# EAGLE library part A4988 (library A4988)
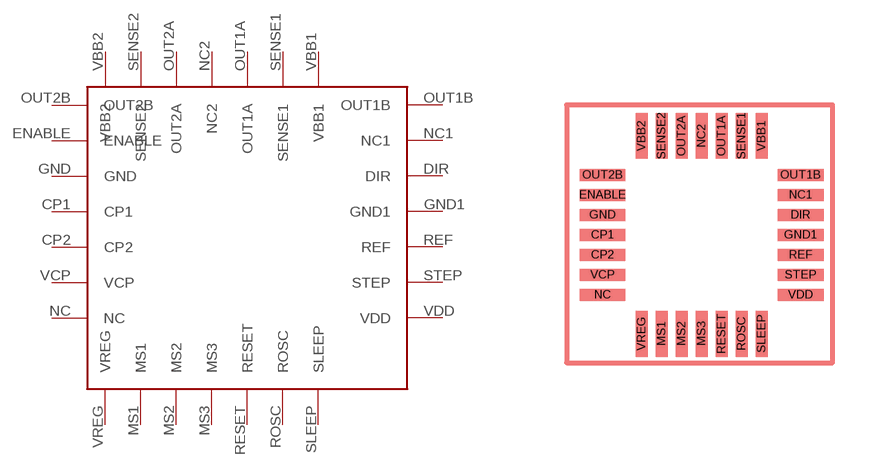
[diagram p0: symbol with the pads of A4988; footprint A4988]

Designator prefix -

## A4988  [A4988]
CP1  CP1
CP2  CP2
DIR  DIR
ENABLE  ENABLE
GND  GND
GND1  GND1
MS1  MS1
MS2  MS2
MS3  MS3
NC  NC
NC1  NC1
NC2  NC2
OUT1A  OUT1A
OUT1B  OUT1B
OUT2A  OUT2A
OUT2B  OUT2B
REF  REF
RESET  RESET
ROSC  ROSC
SENSE1  SENSE1
SENSE2  SENSE2
SLEEP  SLEEP
STEP  STEP
VBB1  VBB1
VBB2  VBB2
VCP  VCP
VDD  VDD
VREG  VREG

## Footprint A4988 (pad centres in mm)
smd 1.15 x 0.3: CP1 0,1.5; CP2 0,1; DIR 4.95,2; ENABLE 0,2.5; GND 0,2; GND1 4.95,1.5; NC 0,0; NC1 4.95,2.5; OUT1B 4.95,3; OUT2B 0,3; REF 4.95,1; STEP 4.95,0.5; VCP 0,0.5; VDD 4.95,0
smd 0.3 x 1.15: MS1 1.475,-0.975; MS2 1.975,-0.975; MS3 2.475,-0.975; NC2 2.475,3.975; OUT1A 2.975,3.975; OUT2A 1.975,3.975; RESET 2.975,-0.975; ROSC 3.475,-0.975; SENSE1 3.475,3.975; SENSE2 1.475,3.975; SLEEP 3.975,-0.975; VBB1 3.975,3.975; VBB2 0.975,3.975; VREG 0.975,-0.975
